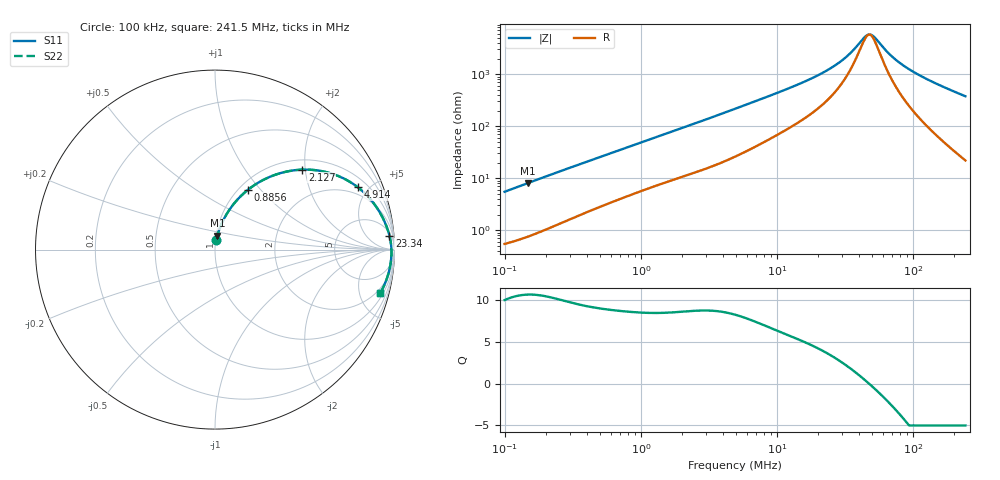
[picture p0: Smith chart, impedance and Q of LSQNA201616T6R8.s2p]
! LSQNA201616T6R8  S-PARAMETER MODEL  ( General Type )
! Model Generated by TAIYO YUDEN Corporation (http://www.ty-top.com)
! Version 2.0
! TAIYO YUDEN Control No. 100810NF25SB-FKC
! Copyright(c) 2007 TAIYO YUDEN CO.,LTD. All Rights Reserved.
! Product Description (link to TY-COMPAS)
! https://ds.yuden.co.jp/TYCOMPAS/or/detail?pn=LSQNA201616T6R8M&u=M
! Products Name : Inductors
! Characteristics :
!  Inductance : 6.8 uH , SRF(min) : 38 MHz , DC Resistance(max) : 0.455 Ohm
!  Rated Current : Saturation :300 mA , Temp Rise : 600 mA (40 degC)
!  Case Size : 2.0 x 1.6 / 0.079 x 0.063 [mm/inch] , Thickness : 1.6 / 0.063 [mm/inch]
!  (Conditions: Temperature = 25 degC , DC Bias Current/Voltage = 0A / 0V)
! External Node Assignments :
!  1  o---GGG---o  2
! GND o---------o GND
! Frequency Range : 0.1MHz  -  241.513628MHz  [ 402 STEP ]
# MHz S RI R 50
! Freq[MHz].  S11 Real  S11 Imag  S21 Real  S21 Imag  S12 Real  S12 Imag  S22 Real  S22 Imag
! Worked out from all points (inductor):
!   401 points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, 100 kHz to 241.5 MHz, reference 50 ohm
!   read as one part in series: L = 8.63 uH near 104 kHz
!   highest Q = 10.7 at 147.6 kHz (marker M1), where L = 8.6 uH
!   self-resonance near 47.49 MHz
!   S11 on the Smith chart (normalised r, x): 100 kHz: 1.01, +0.11; 885.6 kHz: 1.10, +0.86; 2.127 MHz: 1.22, +1.93; 4.914 MHz: 1.52, +4.28; 23.34 MHz: 7, +23; 241.5 MHz: 1.44, -7.51
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0.1  0.00832 0.0537  0.9917 -0.0537  0.9917 -0.0537  0.00832 0.0537
0.147621  0.0136 0.0781  0.9864 -0.0781  0.9864 -0.0781  0.0136 0.0781
0.368674  0.0528 0.1768  0.9472 -0.1768  0.9472 -0.1768  0.0528 0.1768
0.588328  0.1044 0.2546  0.8956 -0.2546  0.8956 -0.2546  0.1044 0.2546
0.885572  0.1834 0.3331  0.8166 -0.3331  0.8166 -0.3331  0.1834 0.3331
1.359207  0.3106 0.4076  0.6894 -0.4076  0.6894 -0.4076  0.3106 0.4076
2.127182  0.4862 0.4454  0.5138 -0.4454  0.5138 -0.4454  0.4862 0.4454
3.140159  0.6469 0.4243  0.3531 -0.4243  0.3531 -0.4243  0.6469 0.4243
4.914404  0.7961 0.347  0.2039 -0.347  0.2039 -0.347  0.7961 0.347
8.644385  0.9047 0.2292  0.0953 -0.2292  0.0953 -0.2292  0.9047 0.2292
18.11814  0.9629 0.1092  0.0371 -0.1092  0.0371 -0.1092  0.9629 0.1092
23.33776  0.9721 0.0772  0.0279 -0.0772  0.0279 -0.0772  0.9721 0.0772
31.86961  0.9792 0.0419  0.0208 -0.0419  0.0208 -0.0419  0.9792 0.0419
43.52056  0.9826 0.00906  0.0174 -0.00906  0.0174 -0.00906  0.9826 0.00906
47.04613  0.983 0.00097  0.017 -0.00097  0.017 -0.00097  0.983 0.00097
48.91461  0.9832 -0.00308  0.0168 0.00308  0.0168 0.00308  0.9832 -0.00308
51.85739  0.9833 -0.00918  0.0167 0.00918  0.0167 0.00918  0.9833 -0.00918
66.79689  0.9827 -0.0363  0.0173 0.0363  0.0173 0.0363  0.9827 -0.0363
82.75365  0.9806 -0.0611  0.0194 0.0611  0.0194 0.0611  0.9806 -0.0611
108.6901  0.9751 -0.0964  0.0249 0.0964  0.0249 0.0964  0.9751 -0.0964
160.4491  0.9588 -0.1579  0.0412 0.1579  0.0412 0.1579  0.9588 -0.1579
241.5136  0.9218 -0.2409  0.0782 0.2409  0.0782 0.2409  0.9218 -0.2409
